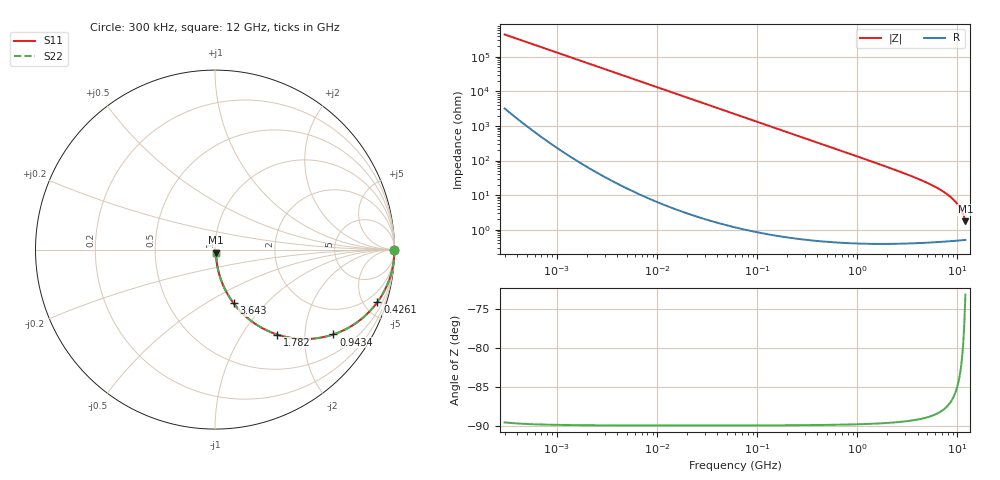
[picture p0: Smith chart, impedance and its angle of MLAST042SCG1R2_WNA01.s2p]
! MLAST042SCG1R2_WNA01  S-PARAMETER MODEL  ( General Type )
! Model Generated by TAIYO YUDEN Corporation (http://www.ty-top.com)
! Version 1.0
! TAIYO YUDEN Control No. 150820
! Copyright(c) 2015 TAIYO YUDEN CO.,LTD. All Rights Reserved.
! Product Description (link to TY-COMPAS)
! https://ds.yuden.co.jp/TYCOMPAS/or/detail?pn=MLAST042SCG1R2AWNA01&u=M
! Products Name : Multilayer Ceramic Capacitors
! Characteristics :
!  Capacitance : 1.2 pF , Rated Voltage : 25V , TCC : CG / C0G
!  Case Size : 0.4 x 0.2 / 0.016 x 0.008 [mm/inch] , Thickness : 0.2 / 0.008 [mm/inch]
!  (Conditions: Temperature = 25 degC , DC Bias Current/Voltage = 0A / 0V)
! External Node Assignments :
!  1  o---| |---o  2
! GND o---------o GND
! Frequency Range : 0.3MHz  -  12000MHz  [ 401 STEP ]
# MHz S RI R 50
! Freq[MHz].  S11 Real  S11 Imag  S21 Real  S21 Imag  S12 Real  S12 Imag  S22 Real  S22 Imag
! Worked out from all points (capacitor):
!   401 points, 300 kHz to 12 GHz, reference 50 ohm
!   read as one part in series: C = 1.2 pF near 316.3 kHz
!   lowest |Z| = 1.75 ohm at 12 GHz (marker M1)
!   S11 on the Smith chart (normalised r, x): 300 kHz: open; 426.1 MHz: 1.01, -6.20; 943.4 MHz: 1.01, -2.79; 1.782 GHz: 1.01, -1.46; 3.643 GHz: 1.01, -0.67; 12 GHz: 1.01, -0.03
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0.3  1 -0.000227  1.7e-06 0.000227  1.7e-06 0.000227  1 -0.000227
1.769972  1 -0.00134  3.24e-06 0.00134  3.24e-06 0.00134  1 -0.00134
10.44266  0.9999 -0.0079  6.62e-05 0.0079  6.62e-05 0.0079  0.9999 -0.0079
60  0.9979 -0.0453  0.00208 0.0453  0.00208 0.0453  0.9979 -0.0453
159.8975  0.9855 -0.1193  0.0145 0.1193  0.0145 0.1193  0.9855 -0.1193
353.9943  0.9327 -0.2499  0.0673 0.2499  0.0673 0.2499  0.9327 -0.2499
426.1204  0.9053 -0.2921  0.0947 0.2921  0.0947 0.2921  0.9053 -0.2921
634.0297  0.8116 -0.39  0.1884 0.39  0.1884 0.39  0.8116 -0.39
943.3804  0.6596 -0.4724  0.3404 0.4724  0.3404 0.4724  0.6596 -0.4724
1296.429  0.5046 -0.498  0.4954 0.498  0.4954 0.498  0.5046 -0.498
1781.601  0.3471 -0.4734  0.6529 0.4734  0.6529 0.4734  0.3471 -0.4734
2088.533  0.2766 -0.4442  0.7234 0.4442  0.7234 0.4442  0.2766 -0.4442
2722.03  0.1794 -0.3795  0.8206 0.3795  0.8206 0.3795  0.1794 -0.3795
3642.919  0.1035 -0.2986  0.8965 0.2986  0.8965 0.2986  0.1035 -0.2986
5868.704  0.0351 -0.1725  0.9649 0.1725  0.9649 0.1725  0.0351 -0.1725
7064.448  0.0214 -0.1287  0.9786 0.1287  0.9786 0.1287  0.0214 -0.1287
8281.503  0.0135 -0.0934  0.9865 0.0934  0.9865 0.0934  0.0135 -0.0934
9207.246  0.0098 -0.0709  0.9902 0.0709  0.9902 0.0709  0.0098 -0.0709
10236.47  0.00725 -0.0489  0.9927 0.0489  0.9927 0.0489  0.00725 -0.0489
10793.46  0.00636 -0.038  0.9936 0.038  0.9936 0.038  0.00636 -0.038
11686.27  0.00549 -0.0219  0.9945 0.0219  0.9945 0.0219  0.00549 -0.0219
12000  0.00532 -0.0166  0.9947 0.0166  0.9947 0.0166  0.00532 -0.0166
